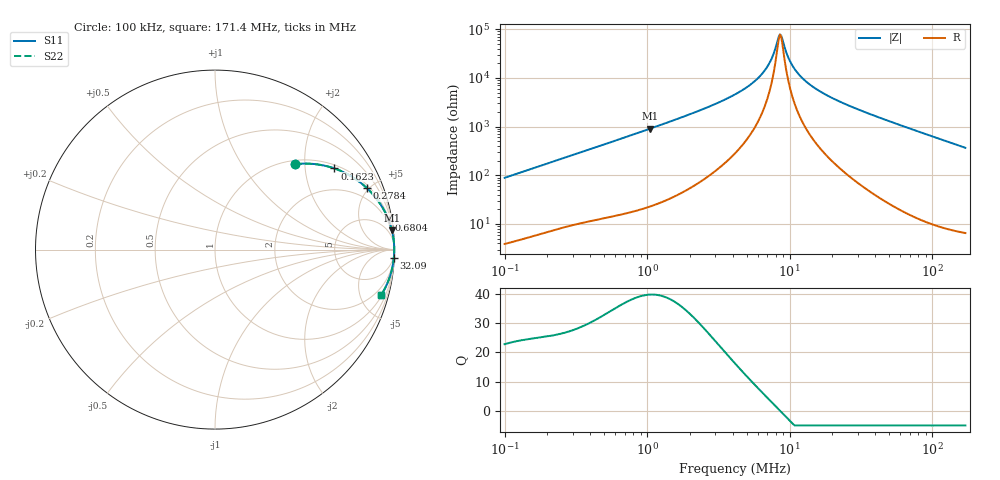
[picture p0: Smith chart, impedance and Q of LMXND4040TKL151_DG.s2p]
! LMXND4040TKL151_DG  S-PARAMETER MODEL  ( General Type )
! Model Generated by TAIYO YUDEN Corporation (http://www.ty-top.com)
! Version 1.0
! TAIYO YUDEN Control No. 191023NI43SB-FBB
! Copyright(c) 2019 TAIYO YUDEN CO.,LTD. All Rights Reserved.
! Product Description (link to TY-COMPAS)
! https://ds.yuden.co.jp/TYCOMPAS/or/detail?pn=LMXND4040TKL151MDG&u=M
! Products Name : Inductors
! Characteristics :
!  Inductance : 150 uH , SRF(min) : 5.5 MHz , DC Resistance(max) : 2.76 Ohm
!  Rated Current : Saturation :340 mA , Temp Rise : 220 mA
!  Case Size : 4.0 x 4.0 / 0.157 x 0.157 [mm/inch] , Thickness : 1.8 / 0.071 [mm/inch]
!  (Conditions: Temperature = 25 degC , DC Bias Current/Voltage = 0A / 0V)
! External Node Assignments :
!  1  o---GGG---o  2
! GND o---------o GND
! Frequency Range : 0.1MHz  -  171.398534MHz  [ 402 STEP ]
# MHz S RI R 50
! Freq[MHz].  S11 Real  S11 Imag  S21 Real  S21 Imag  S12 Real  S12 Imag  S22 Real  S22 Imag
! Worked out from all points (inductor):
!   401 points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, 100 kHz to 171.4 MHz, reference 50 ohm
!   read as one part in series: L = 141 uH near 103.8 kHz
!   highest Q = 39.7 at 1.044 MHz (marker M1), where L = 138 uH
!   self-resonance near 8.557 MHz
!   S11 on the Smith chart (normalised r, x): 100 kHz: 1.08, +1.78; 162.3 kHz: 1.12, +2.86; 278.4 kHz: 1.18, +4.85; 680.4 kHz: 1, +12; 32.09 MHz: 2, -42; 171.4 MHz: 1.13, -7.35
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0.1  0.4439 0.4753  0.5561 -0.4753  0.5561 -0.4753  0.4439 0.4753
0.16226  0.6657 0.452  0.3343 -0.452  0.3343 -0.452  0.6657 0.452
0.278404  0.8458 0.3431  0.1542 -0.3431  0.1542 -0.3431  0.8458 0.3431
0.348094  0.893 0.2922  0.107 -0.2922  0.107 -0.2922  0.893 0.2922
0.680388  0.9675 0.1642  0.0325 -0.1642  0.0325 -0.1642  0.9675 0.1642
1.044028  0.9853 0.1086  0.0147 -0.1086  0.0147 -0.1086  0.9853 0.1086
1.211692  0.9888 0.0935  0.0112 -0.0935  0.0112 -0.0935  0.9888 0.0935
4.140031  0.9982 0.0217  0.00182 -0.0217  0.00182 -0.0217  0.9982 0.0217
5.473673  0.9985 0.0127  0.00146 -0.0127  0.00146 -0.0127  0.9985 0.0127
6.593697  0.9987 0.00731  0.00134 -0.00731  0.00134 -0.00731  0.9987 0.00731
7.372913  0.9987 0.00419  0.0013 -0.00419  0.0013 -0.00419  0.9987 0.00419
8.244213  0.9987 0.00113  0.00128 -0.00113  0.00128 -0.00113  0.9987 0.00113
8.556955  0.9987 0.000116  0.00127 -0.000116  0.00127 -0.000116  0.9987 0.000116
8.881561  0.9987 -0.000899  0.00127 0.000899  0.00127 0.000899  0.9987 -0.000899
9.747974  0.9987 -0.00345  0.00128 0.00345  0.00128 0.00345  0.9987 -0.00345
10.69891  0.9987 -0.00602  0.00131 0.00602  0.00131 0.00602  0.9987 -0.00602
12.18806  0.9986 -0.00972  0.00136 0.00972  0.00136 0.00972  0.9986 -0.00972
14.41119  0.9985 -0.0147  0.00149 0.0147  0.00149 0.0147  0.9985 -0.0147
19.7763  0.9981 -0.0254  0.00194 0.0254  0.00194 0.0254  0.9981 -0.0254
32.08895  0.9964 -0.0471  0.0036 0.0471  0.0036 0.0471  0.9964 -0.0471
50.16444  0.9925 -0.0767  0.00748 0.0767  0.00748 0.0767  0.9925 -0.0767
171.3985  0.9273 -0.2509  0.0727 0.2509  0.0727 0.2509  0.9273 -0.2509
